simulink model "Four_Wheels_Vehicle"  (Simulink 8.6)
settings: Solver=ode45  StartTime=0.0  StopTime=20  RelTol=1e-3
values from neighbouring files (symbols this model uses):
  beta = 1    [Vehicle_Parameters.m]
  g = 9.81    [Vehicle_Parameters.m]
  H_CoG = 0.700    (= 0.7)    [Vehicle_Parameters.m]
  Hearo = 0.750    (= 0.75)    [Vehicle_Parameters.m]
  Iz = 2480    [Vehicle_Parameters.m]
  Jw = 2.166    [Vehicle_Parameters.m]
  L = 10    [Vehicle_Parameters.m]
  Lf = 1.180    (= 1.18)    [Vehicle_Parameters.m]
  Lr = 1.770    (= 1.77)    [Vehicle_Parameters.m]
  Lw = 1.880    (= 1.88)    [Vehicle_Parameters.m]
  m = 1500    [Vehicle_Parameters.m]
  miu = 0.85    [Vehicle_Parameters.m]
  reff = 0.380    (= 0.38)    [Vehicle_Parameters.m]
undefined symbols (not defined in the file or in its folder): DiscIntNeverNeededParam, Init, Ki, Kp, LowerLimit, sigbuilder_block, Ts, UpperLimit
libraries: simulink x15, powerlib_extras x3
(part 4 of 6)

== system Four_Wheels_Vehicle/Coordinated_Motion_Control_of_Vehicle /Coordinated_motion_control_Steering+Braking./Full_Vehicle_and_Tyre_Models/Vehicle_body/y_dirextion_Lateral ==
  note: y_dirextion_Lateral
  Fx_FL : Inport
  Fx_FR : Inport  Port=2
  Fy_FL : Inport  Port=3
  Fy_FR : Inport  Port=4
  Fy_RL : Inport  Port=5
  Fy_RR : Inport  Port=6
  Steering_Ang. : Inport  Port=7
  yaw_rate : Inport  Port=8
  x_Vel : Inport  Port=9
  1/m : Gain  Gain=1/1750
  Add1 : Sum
  Add12 : Sum
  Add15 : Sum  Inputs=++++
  Add2 : Sum  Inputs=+-
  Product1 : Product
  Product13 : Product
  Product3 : Product
  Vx0 : Integrator  UpperSaturationLimit=50/3.6  LowerSaturationLimit=eps
  cos_deltaw2 : Fcn  Expr=cos(u)
  sin_deltaw2 : Fcn  Expr=sin(u)
  y_Vel : Outport
  y total force : Outport  Port=2
  dy : Outport  Port=3
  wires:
  Steering_Ang./1 -> sin_deltaw2/1, cos_deltaw2/1
  Add12/1 -> Product13/1
  sin_deltaw2/1 -> Product13/2
  Add15/1 -> 1/m/1, y total force/1
  1/m/1 -> Add2/1
  Vx0/1 -> y_Vel/1
  Add1/1 -> Product1/1
  cos_deltaw2/1 -> Product1/2
  yaw_rate/1 -> Product3/1
  x_Vel/1 -> Product3/2
  Product3/1 -> Add2/2
  Fy_FL/1 -> Add1/1
  Fy_FR/1 -> Add1/2
  Fx_FL/1 -> Add12/1
  Fx_FR/1 -> Add12/2
  Product1/1 -> Add15/2
  Product13/1 -> Add15/1
  Fy_RR/1 -> Add15/4
  Fy_RL/1 -> Add15/3
  Add2/1 -> dy/1, Vx0/1

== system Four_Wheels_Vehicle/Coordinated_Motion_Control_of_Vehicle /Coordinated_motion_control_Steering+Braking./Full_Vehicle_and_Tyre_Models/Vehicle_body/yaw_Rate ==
  note: yaw_Rate_and_z_torque
  Fx_FL : Inport
  Fx_FR : Inport  Port=2
  Fy_FL : Inport  Port=3
  Fy_FR : Inport  Port=4
  Fx_RL : Inport  Port=5
  Fx_RR : Inport  Port=6
  Fy_RL : Inport  Port=7
  Fy_RR : Inport  Port=8
  Steering_Ang. : Inport  Port=9
  1/Iz : Gain  Gain=1/Iz
  Add1 : Sum  Inputs=-+
  Add10 : Sum  Inputs=+++++-
  Add2 : Sum
  Add3 : Sum  Inputs=-+
  Add4 : Sum
  Add5 : Sum  Inputs=-+
  Add6 : Sum
  Integrator1 : Integrator  InitialCondition=eps  UpperSaturationLimit=50/3.6  LowerSaturationLimit=eps  ShowSaturationPort=on
  Lf : Constant  Value=Lf
  Lr : Constant  Value=Lr
  Lw/2 : Constant  Value=Lw/2
  Product{1..9,13} (10 alike) : Product
  Stop Simulation1 : Stop
  cosdeltaw1 : Fcn  Expr=cos(u)
  sindeltaw1 : Fcn  Expr=sin(u)
  yaw_rate : Outport
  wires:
  Steering_Ang./1 -> cosdeltaw1/1, sindeltaw1/1
  Add4/1 -> Product1/1
  sindeltaw1/1 -> Product6/1, Product1/2
  Lf/1 -> Product3/2, Product13/1
  Add1/1 -> Product4/1
  cosdeltaw1/1 -> Product7/2, Product4/2
  Lw/2/1 -> Product5/2, Product2/2, Product9/2
  Lr/1 -> Product8/2
  Product3/1 -> Add10/1
  1/Iz/1 -> Integrator1/1
  Integrator1/1 -> yaw_rate/1
  Integrator1/2 -> Stop Simulation1/1
  Product1/1 -> Product3/1
  Product4/1 -> Product2/1
  Add2/1 -> Product7/1
  Add5/1 -> Product9/1
  Add6/1 -> Product8/1
  Product13/1 -> Add10/2
  Product7/1 -> Product13/2
  Product2/1 -> Add10/3
  Product8/1 -> Add10/6
  Product9/1 -> Add10/5
  Product5/1 -> Add10/4
  Product6/1 -> Product5/1
  Add3/1 -> Product6/2
  Add10/1 -> 1/Iz/1
  Fy_FR/1 -> Add2/2, Add3/1
  Fy_FL/1 -> Add3/2, Add2/1
  Fx_FL/1 -> Add4/1, Add1/1
  Fx_FR/1 -> Add4/2, Add1/2
  Fx_RL/1 -> Add5/1
  Fx_RR/1 -> Add5/2
  Fy_RL/1 -> Add6/1
  Fy_RR/1 -> Add6/2

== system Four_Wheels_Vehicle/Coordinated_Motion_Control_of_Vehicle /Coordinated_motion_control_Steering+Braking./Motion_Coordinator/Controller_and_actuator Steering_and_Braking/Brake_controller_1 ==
  Reference_Sideslip_1 : Inport
  Feedback_Sideslip_1 : Inport  Port=2
  Add1 : Sum
  Brake_Actuator_1 : Subsystem
  Brake_controller_1 : Subsystem
  Ramp : simulink/Sources/Ramp  slope=3  start=1  X0=0
  Sideslip_angle : Scope  NumInputPorts=2
  x_seitch2 : ManualSwitch  CurrentSetting=0
  Mzc_1 : Outport
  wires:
  Brake_Actuator_1/1(output) -> x_seitch2/2
  Ramp/1 -> x_seitch2/1
  Feedback_Sideslip_1/1 -> Sideslip_angle/2, Brake_controller_1/2(Feedback)
  Brake_controller_1/2(Sideslip_Ang1) -> Brake_Actuator_1/1(input)
  Reference_Sideslip_1/1 -> Add1/1, Sideslip_angle/1, Brake_controller_1/1(Reference)
  Add1/1 -> Mzc_1/1
  x_seitch2/1 -> Add1/2

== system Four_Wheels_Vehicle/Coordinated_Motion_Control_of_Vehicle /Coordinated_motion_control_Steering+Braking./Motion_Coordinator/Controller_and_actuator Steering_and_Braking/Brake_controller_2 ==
  Reference_Sideslip_2 : Inport
  Feedback_Sideslip_2 : Inport  Port=2
  Add1 : Sum
  Brake_Actuator_2 : Subsystem
  Brake_controller_2 : Subsystem
  Ramp : simulink/Sources/Ramp  slope=3  start=1  X0=0
  Sideslip_angle : Scope  NumInputPorts=2
  x_seitch2 : ManualSwitch  CurrentSetting=0
  Mzc_2 : Outport
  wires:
  x_seitch2/1 -> Add1/2
  Add1/1 -> Mzc_2/1
  Reference_Sideslip_2/1 -> Brake_controller_2/1(Reference), Sideslip_angle/1, Add1/1
  Brake_controller_2/2(Sideslip_Ang1) -> Brake_Actuator_2/1(input)
  Feedback_Sideslip_2/1 -> Brake_controller_2/2(Feedback), Sideslip_angle/2
  Ramp/1 -> x_seitch2/1
  Brake_Actuator_2/1(output) -> x_seitch2/2

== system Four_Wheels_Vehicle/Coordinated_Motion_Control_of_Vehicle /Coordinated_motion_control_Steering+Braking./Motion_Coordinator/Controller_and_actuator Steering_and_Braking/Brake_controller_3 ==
  Reference_Sideslip_3 : Inport
  Feedback_Sideslip_3 : Inport  Port=2
  Add1 : Sum
  Brake_Actuator_3 : Subsystem
  Brake_controller_3 : Subsystem
  Ramp : simulink/Sources/Ramp  slope=3  start=1  X0=0
  Sideslip_angle : Scope  NumInputPorts=2
  x_seitch2 : ManualSwitch  CurrentSetting=0
  Mzc_3 : Outport
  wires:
  Brake_Actuator_3/1(output) -> x_seitch2/2
  Ramp/1 -> x_seitch2/1
  Feedback_Sideslip_3/1 -> Sideslip_angle/2, Brake_controller_3/2(Feedback)
  Brake_controller_3/2(Sideslip_Ang1) -> Brake_Actuator_3/1(input)
  Reference_Sideslip_3/1 -> Add1/1, Sideslip_angle/1, Brake_controller_3/1(Reference)
  Add1/1 -> Mzc_3/1
  x_seitch2/1 -> Add1/2

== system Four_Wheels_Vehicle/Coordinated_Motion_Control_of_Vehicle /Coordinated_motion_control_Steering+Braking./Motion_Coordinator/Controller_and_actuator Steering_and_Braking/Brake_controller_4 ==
  Reference_Sideslip_4 : Inport
  Feedback_Sideslip_4 : Inport  Port=2
  Add1 : Sum
  Brake_Actuator_4 : Subsystem
  Brake_controller_4 : Subsystem
  Ramp : simulink/Sources/Ramp  slope=3  start=1  X0=0
  Sideslip_angle : Scope  NumInputPorts=2
  x_seitch2 : ManualSwitch  CurrentSetting=0
  Mzc_4 : Outport
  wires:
  x_seitch2/1 -> Add1/2
  Add1/1 -> Mzc_4/1
  Reference_Sideslip_4/1 -> Brake_controller_4/1(Reference), Sideslip_angle/1, Add1/1
  Brake_controller_4/2(Sideslip_Ang1) -> Brake_Actuator_4/1(input)
  Feedback_Sideslip_4/1 -> Brake_controller_4/2(Feedback), Sideslip_angle/2
  Ramp/1 -> x_seitch2/1
  Brake_Actuator_4/1(output) -> x_seitch2/2

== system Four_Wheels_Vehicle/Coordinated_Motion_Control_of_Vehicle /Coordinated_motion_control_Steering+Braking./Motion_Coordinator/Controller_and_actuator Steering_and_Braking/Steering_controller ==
  StteringAng : Inport
  Reference_Steering : Inport  Port=2
  Feedback_Steering : Inport  Port=3
  Add : Sum
  Steering_Actuator : Subsystem
  Steering_controller : Subsystem
  x_seitch1 : ManualSwitch  CurrentSetting=0
  yaw_comparsion : Scope  NumInputPorts=2
  f : Outport
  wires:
  Add/1 -> f/1
  Feedback_Steering/1 -> yaw_comparsion/2, Steering_controller/2(Feedback)
  Steering_Actuator/1(output) -> x_seitch1/2
  Steering_controller/2(Steering_Ang1) -> Steering_Actuator/1(input)
  x_seitch1/1 -> Add/2
  StteringAng/1 -> Add/1
  Reference_Steering/1 -> x_seitch1/1, Steering_controller/1(Reference), yaw_comparsion/1

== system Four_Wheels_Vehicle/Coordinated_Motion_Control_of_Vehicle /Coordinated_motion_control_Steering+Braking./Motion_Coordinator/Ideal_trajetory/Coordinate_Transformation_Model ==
  note: vehicle heading
  delta_steer (rad) : Inport
  v_x (m/s) : Inport  Port=2
  1/L : Gain  Gain=1/L
  Beta : Scope
  Beta1 : Scope
  Divide : Product  Inputs=*/
  Gain : Gain  Gain=L/2
  Gain1 : Gain  Gain=0.1
  Gain2 : Gain  Gain=0.1
  Gain4 : Gain  Gain=0.345
  Ground : Ground
  Integrator : Integrator
  Integrator1 : Integrator  LimitOutput=on  UpperSaturationLimit=0
  Integrator2 : Integrator
  Product{,1,3..4} (4 alike) : Product
  Sideslip_angle : Scope
  Subtract : Sum  Inputs=+-
  Sum : Sum  Inputs=|+-
  Sum1 : Sum  Inputs=|++
  Terminator : Terminator
  Trigonometric Function : Trigonometry  Operator=cos
  Trigonometric Function1 : Trigonometry
  Trigonometric Function2 : Trigonometry  Operator=atan
  Trigonometric Function3 : Trigonometry  Operator=tan
  steerVsYawrate1 : Scope  NumInputPorts=3
  steerVsYawrate2 : Scope  NumInputPorts=3
  yaw_rate : Product
  X-position : Outport
  Y-position : Outport  Port=2
  yaw_Rate : Outport  Port=3
  Sideslip_beta : Outport  Port=4
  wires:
  Subtract/1 -> Beta/1
  Gain4/1 -> Divide/1, Integrator1/1, steerVsYawrate2/3
  Trigonometric Function2/1 -> Subtract/1, Sideslip_beta/1, Sideslip_angle/1
  Gain2/1 -> Integrator2/1
  Gain1/1 -> Trigonometric Function1/1, steerVsYawrate1/3, Trigonometric Function/1
  delta_steer (rad)/1 -> yaw_rate/2
  Divide/1 -> Trigonometric Function2/1
  Trigonometric Function3/1 -> Terminator/1
  Ground/1 -> Trigonometric Function3/1
  Product4/1 -> Sum1/2
  Product3/1 -> Sum/2
  Gain/1 -> Product4/1, Product3/1  "L/2*psi-dot"
  Sum1/1 -> Gain4/1  "v_Y (m/s)"
  Sum/1 -> Divide/2, Integrator/1, steerVsYawrate2/2  "v_X (m/s)"
  1/L/1 -> yaw_rate/1  "v_x / L"
  yaw_rate/1 -> Gain2/1, yaw_Rate/1, Subtract/2, Beta1/1, Gain/1, steerVsYawrate2/1
  v_x (m/s)/1 -> 1/L/1, Product1/1, Product/1  "v_x (m/s)"
  Integrator1/1 -> Y-position/1, steerVsYawrate1/2
  Integrator/1 -> X-position/1, steerVsYawrate1/1
  Integrator2/1 -> Gain1/1  "yaw_heading (rad)"
  Trigonometric Function1/1 -> Product3/2, Product/2  "sin(psi)"
  Trigonometric Function/1 -> Product4/2, Product1/2  "cos(psi)"
  Product1/1 -> Sum/1
  Product/1 -> Sum1/1

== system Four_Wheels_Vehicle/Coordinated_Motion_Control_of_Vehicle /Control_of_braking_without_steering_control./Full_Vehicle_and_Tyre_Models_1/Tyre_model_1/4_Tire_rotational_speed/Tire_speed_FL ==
  Tb_FL_1 : Inport
  Td_FL_1 : Inport  Port=2
  Fx_FL_1 : Inport  Port=3
  1/Jw : Gain  Gain=1/Jw
  Add22 : Sum  Inputs=-+
  Add23 : Sum  Inputs=+-
  Product27 : Product
  Stop Simulation5 : Stop
  Vx0 : Integrator  InitialCondition=14.3  UpperSaturationLimit=50/3.6  LowerSaturationLimit=eps  ShowSaturationPort=on
  reff : Constant  Value=reff
  Omega_FL_1 : Outport
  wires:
  Fx_FL_1/1 -> Product27/1
  Vx0/2 -> Stop Simulation5/1
  Vx0/1 -> Omega_FL_1/1
  Add23/1 -> 1/Jw/1
  Add22/1 -> Add23/1
  Product27/1 -> Add23/2
  reff/1 -> Product27/2
  Td_FL_1/1 -> Add22/2
  Tb_FL_1/1 -> Add22/1
  1/Jw/1 -> Vx0/1

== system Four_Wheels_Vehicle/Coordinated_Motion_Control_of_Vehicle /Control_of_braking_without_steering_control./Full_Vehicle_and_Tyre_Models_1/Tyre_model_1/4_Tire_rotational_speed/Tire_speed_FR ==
  Tb_FR_1 : Inport
  Td_FR_1 : Inport  Port=2
  Fx_FR_1 : Inport  Port=3
  1/Jw : Gain  Gain=1/Jw
  Add1 : Sum  Inputs=+-
  Add24 : Sum  Inputs=-+
  Product1 : Product
  Stop Simulation6 : Stop
  Vx1 : Integrator  InitialCondition=14.3  UpperSaturationLimit=50/3.6  LowerSaturationLimit=eps  ShowSaturationPort=on
  reff : Constant  Value=reff
  Omega_FR_1 : Outport
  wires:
  Vx1/1 -> Omega_FR_1/1
  Vx1/2 -> Stop Simulation6/1
  Fx_FR_1/1 -> Product1/1
  reff/1 -> Product1/2
  Tb_FR_1/1 -> Add24/1
  Td_FR_1/1 -> Add24/2
  Add24/1 -> Add1/1
  1/Jw/1 -> Vx1/1
  Add1/1 -> 1/Jw/1
  Product1/1 -> Add1/2

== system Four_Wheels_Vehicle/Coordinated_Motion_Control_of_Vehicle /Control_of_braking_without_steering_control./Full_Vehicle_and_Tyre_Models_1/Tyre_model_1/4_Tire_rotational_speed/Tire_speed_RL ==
  Tb_RL_1 : Inport
  Td_RL_1 : Inport  Port=2
  Fx_RL_1 : Inport  Port=3
  1/Jw : Gain  Gain=1/Jw
  Add2 : Sum  Inputs=--
  Add22 : Sum  Inputs=-+
  Product2 : Product
  Stop Simulation7 : Stop
  Vx2 : Integrator  InitialCondition=14.3  UpperSaturationLimit=50/3.6  LowerSaturationLimit=eps  ShowSaturationPort=on
  reff : Constant  Value=reff
  Omega_RL_1 : Outport
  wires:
  Td_RL_1/1 -> Add22/2
  Tb_RL_1/1 -> Add22/1
  Add22/1 -> Add2/1
  Add2/1 -> 1/Jw/1
  Product2/1 -> Add2/2
  reff/1 -> Product2/2
  Vx2/1 -> Omega_RL_1/1
  Vx2/2 -> Stop Simulation7/1
  1/Jw/1 -> Vx2/1
  Fx_RL_1/1 -> Product2/1

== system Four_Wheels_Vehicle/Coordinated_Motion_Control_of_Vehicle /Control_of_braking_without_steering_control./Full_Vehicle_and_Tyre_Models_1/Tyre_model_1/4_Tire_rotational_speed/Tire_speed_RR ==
  Tb_RR_1 : Inport
  Td_RR_1 : Inport  Port=2
  Fx_RR_1 : Inport  Port=3
  1/Jw : Gain  Gain=1/Jw
  Add22 : Sum  Inputs=-+
  Add3 : Sum  Inputs=--
  Product3 : Product
  Stop Simulation8 : Stop
  Vx3 : Integrator  InitialCondition=14.3  UpperSaturationLimit=50/3.6  LowerSaturationLimit=eps  ShowSaturationPort=on
  reff : Constant  Value=reff
  Omega_RR_1 : Outport
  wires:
  Td_RR_1/1 -> Add22/2
  Tb_RR_1/1 -> Add22/1
  Add22/1 -> Add3/1
  Product3/1 -> Add3/2
  Fx_RR_1/1 -> Product3/1
  reff/1 -> Product3/2
  1/Jw/1 -> Vx3/1
  Add3/1 -> 1/Jw/1
  Vx3/2 -> Stop Simulation8/1
  Vx3/1 -> Omega_RR_1/1

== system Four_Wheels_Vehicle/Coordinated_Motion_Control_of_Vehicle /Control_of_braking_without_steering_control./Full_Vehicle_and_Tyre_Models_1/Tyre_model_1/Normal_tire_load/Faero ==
  note: Air Drag Faero
  Vx : Inport
  AirDragConst1 : Inport  Port=2
  FrontalArea1 : Inport  Port=3
  Airdensity : Inport  Port=4
  windVelocity : Inport  Port=5
  Add : Sum
  Constant : Constant  Value=0.5
  Math Function : Math  Operator=square
  Product : Product  Inputs=5
  Faero : Outport
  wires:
  Vx/1 -> Add/2
  Airdensity/1 -> Product/3
  AirDragConst1/1 -> Product/1
  Product/1 -> Faero/1
  Math Function/1 -> Product/5
  Add/1 -> Math Function/1
  windVelocity/1 -> Add/1
  Constant/1 -> Product/4
  FrontalArea1/1 -> Product/2

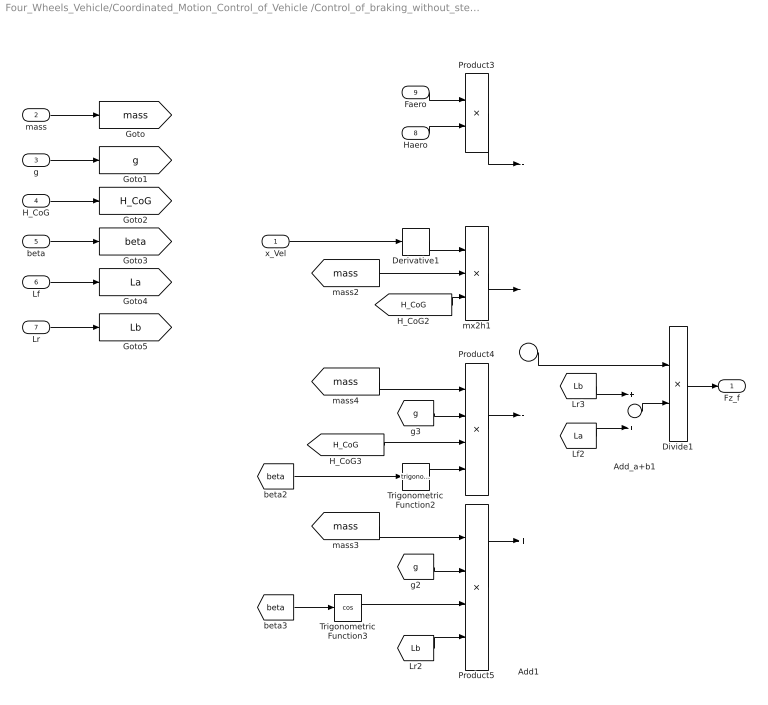
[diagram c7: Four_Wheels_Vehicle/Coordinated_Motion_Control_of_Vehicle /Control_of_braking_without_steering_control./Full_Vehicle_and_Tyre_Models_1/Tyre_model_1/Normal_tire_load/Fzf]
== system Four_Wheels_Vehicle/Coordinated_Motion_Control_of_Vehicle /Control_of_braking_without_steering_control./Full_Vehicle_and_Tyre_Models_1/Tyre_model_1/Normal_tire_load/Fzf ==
  x_Vel : Inport
  mass : Inport  Port=2
  g : Inport  Port=3
  H_CoG : Inport  Port=4
  beta : Inport  Port=5
  Lf : Inport  Port=6
  Lr : Inport  Port=7
  Haero : Inport  Port=8
  Faero : Inport  Port=9
  Add1 : Sum  Inputs=---+
  Add_a+b1 : Sum
  Derivative1 : Derivative
  Divide1 : Product  Inputs=*/
  Product3 : Product
  Product4 : Product  Inputs=4
  Product5 : Product  Inputs=4
  Trigonometric Function2 : Trigonometry
  Trigonometric Function3 : Trigonometry  Operator=cos
  mx2h1 : Product  Inputs=3
  Fz_f : Outport
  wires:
  Lf/1 -> [La]
  mass/1 -> [mass]
  Haero/1 -> Product3/2
  Faero/1 -> Product3/1
  Lr/1 -> [Lb]
  beta/1 -> [beta]
  H_CoG/1 -> [H_CoG]
  g/1 -> [g]
  [g] -> Product5/2
  [mass] -> mx2h1/2
  [g] -> Product4/2
  [mass] -> Product4/1
  x_Vel/1 -> Derivative1/1
  Divide1/1 -> Fz_f/1
  Add_a+b1/1 -> Divide1/2
  Add1/1 -> Divide1/1
  Product5/1 -> Add1/4
  Product4/1 -> Add1/3
  mx2h1/1 -> Add1/2
  Product3/1 -> Add1/1
  [La] -> Add_a+b1/2
  [Lb] -> Add_a+b1/1
  [Lb] -> Product5/4
  Trigonometric Function3/1 -> Product5/3
  [mass] -> Product5/1
  Trigonometric Function2/1 -> Product4/4
  [H_CoG] -> Product4/3
  [beta] -> Trigonometric Function3/1
  [beta] -> Trigonometric Function2/1
  [H_CoG] -> mx2h1/3
  Derivative1/1 -> mx2h1/1

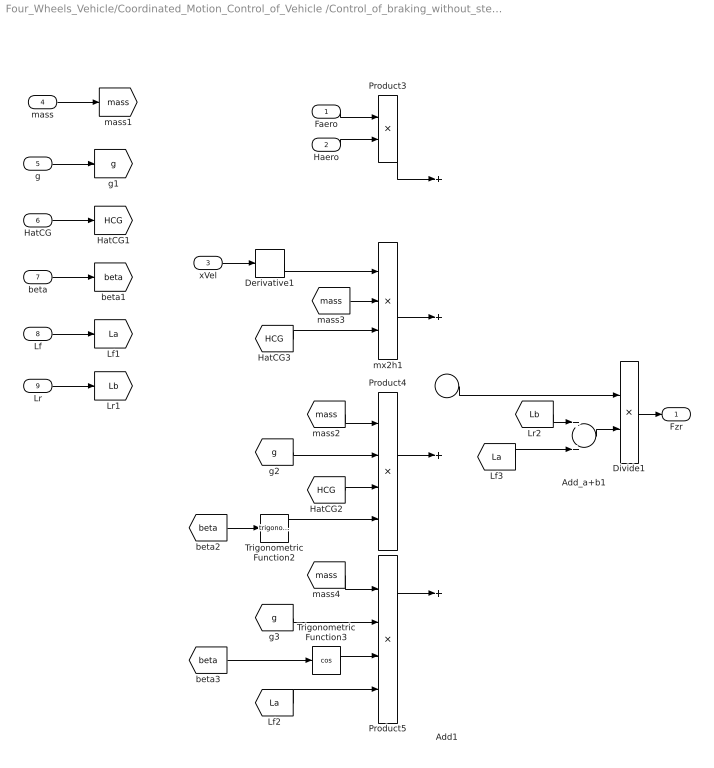
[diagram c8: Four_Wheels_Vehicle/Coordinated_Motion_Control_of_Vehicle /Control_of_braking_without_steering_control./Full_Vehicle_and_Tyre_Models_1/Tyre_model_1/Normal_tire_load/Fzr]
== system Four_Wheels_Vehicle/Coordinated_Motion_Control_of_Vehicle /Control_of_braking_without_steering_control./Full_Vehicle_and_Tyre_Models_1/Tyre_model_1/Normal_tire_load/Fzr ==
  Faero : Inport
  Haero : Inport  Port=2
  xVel : Inport  Port=3
  mass : Inport  Port=4
  g : Inport  Port=5
  HatCG : Inport  Port=6
  beta : Inport  Port=7
  Lf : Inport  Port=8
  Lr : Inport  Port=9
  Add1 : Sum  Inputs=++++
  Add_a+b1 : Sum
  Derivative1 : Derivative
  Divide1 : Product  Inputs=*/
  Product3 : Product
  Product4 : Product  Inputs=4
  Product5 : Product  Inputs=4
  Trigonometric Function2 : Trigonometry
  Trigonometric Function3 : Trigonometry  Operator=cos
  mx2h1 : Product  Inputs=3
  Fzr : Outport
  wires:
  Faero/1 -> Product3/1
  Haero/1 -> Product3/2
  Derivative1/1 -> mx2h1/1
  [HCG] -> mx2h1/3
  [beta] -> Trigonometric Function2/1
  [beta] -> Trigonometric Function3/1
  [HCG] -> Product4/3
  Trigonometric Function2/1 -> Product4/4
  [mass] -> Product5/1
  Trigonometric Function3/1 -> Product5/3
  [La] -> Product5/4
  [Lb] -> Add_a+b1/1
  [La] -> Add_a+b1/2
  Product3/1 -> Add1/1
  mx2h1/1 -> Add1/2
  Product4/1 -> Add1/3
  Product5/1 -> Add1/4
  Add1/1 -> Divide1/1
  Add_a+b1/1 -> Divide1/2
  Divide1/1 -> Fzr/1
  xVel/1 -> Derivative1/1
  mass/1 -> [mass]
  [mass] -> Product4/1
  g/1 -> [g]
  [g] -> Product4/2
  [mass] -> mx2h1/2
  [g] -> Product5/2
  HatCG/1 -> [HCG]
  beta/1 -> [beta]
  Lf/1 -> [La]
  Lr/1 -> [Lb]

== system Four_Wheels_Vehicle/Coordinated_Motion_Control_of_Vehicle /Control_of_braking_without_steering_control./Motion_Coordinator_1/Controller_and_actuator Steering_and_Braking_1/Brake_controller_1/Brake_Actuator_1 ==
  input : Inport
  Actuator : Subsystem
  Cut_off_frequency : Constant  Value=10  SampleTime=-1
  output : Outport
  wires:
  Cut_off_frequency/1 -> Actuator/2(fre)
  Actuator/1(out) -> output/1
  input/1 -> Actuator/1(In1)

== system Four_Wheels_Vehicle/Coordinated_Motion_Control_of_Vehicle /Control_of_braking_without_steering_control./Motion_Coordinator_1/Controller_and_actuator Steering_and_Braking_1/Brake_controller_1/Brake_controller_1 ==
  Reference : Inport
  Feedback : Inport  Port=2
  Controller : Subsystem  AncestorBlock=|  DialogController=POWERSYS.PowerSysDialog
      | powerlib_extras/Discrete 
      | Control Blocks/Discrete
      | PI Controller
  Controller1 : Subsystem  AncestorBlock=|  DialogController=POWERSYS.PowerSysDialog
      | powerlib_extras/Discrete 
      | Control Blocks/Discrete
      | PI Controller
  Scope : Scope
  Scope1 : Scope
  Scope2 : Scope  NumInputPorts=2
  Sum1 : Sum  Inputs=-+
  Sum2 : Sum
  Sideslip_Ang : Outport
  Sideslip_Ang1 : Outport  Port=2
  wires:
  Sum2/1 -> Sideslip_Ang1/1, Scope2/2
  Reference/1 -> Sum1/2, Controller1/1(Error)
  Controller1/1(Out) -> Sum2/2
  Feedback/1 -> Sum1/1
  Sum1/1 -> Scope/1, Controller/1(Error)
  Controller/1(Out) -> Sideslip_Ang/1, Scope2/1, Sum2/1, Scope1/1

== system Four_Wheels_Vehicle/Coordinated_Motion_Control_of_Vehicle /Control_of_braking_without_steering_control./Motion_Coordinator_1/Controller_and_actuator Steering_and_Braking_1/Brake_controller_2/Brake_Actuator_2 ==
  input : Inport
  Actuator : Subsystem
  Cut_off_frequency : Constant  Value=10  SampleTime=-1
  output : Outport
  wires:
  input/1 -> Actuator/1(In1)
  Actuator/1(out) -> output/1
  Cut_off_frequency/1 -> Actuator/2(fre)

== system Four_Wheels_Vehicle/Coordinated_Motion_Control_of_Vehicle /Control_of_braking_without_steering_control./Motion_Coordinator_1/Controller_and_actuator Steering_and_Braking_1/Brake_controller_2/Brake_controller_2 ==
  Reference : Inport
  Feedback : Inport  Port=2
  Controller : Subsystem  AncestorBlock=|  DialogController=POWERSYS.PowerSysDialog
      | powerlib_extras/Discrete 
      | Control Blocks/Discrete
      | PI Controller
  Controller1 : Subsystem  AncestorBlock=|  DialogController=POWERSYS.PowerSysDialog
      | powerlib_extras/Discrete 
      | Control Blocks/Discrete
      | PI Controller
  Scope : Scope
  Scope1 : Scope
  Scope2 : Scope  NumInputPorts=2
  Sum1 : Sum  Inputs=-+
  Sum2 : Sum
  Sideslip_Ang : Outport
  Sideslip_Ang1 : Outport  Port=2
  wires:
  Controller/1(Out) -> Scope1/1, Sum2/1, Scope2/1, Sideslip_Ang/1
  Sum1/1 -> Controller/1(Error), Scope/1
  Feedback/1 -> Sum1/1
  Controller1/1(Out) -> Sum2/2
  Reference/1 -> Controller1/1(Error), Sum1/2
  Sum2/1 -> Scope2/2, Sideslip_Ang1/1

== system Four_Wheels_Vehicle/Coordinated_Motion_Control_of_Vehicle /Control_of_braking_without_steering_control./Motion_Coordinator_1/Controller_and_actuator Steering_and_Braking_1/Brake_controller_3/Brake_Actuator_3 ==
  input : Inport
  Actuator : Subsystem
  Cut_off_frequency : Constant  Value=10  SampleTime=-1
  output : Outport
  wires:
  Cut_off_frequency/1 -> Actuator/2(fre)
  Actuator/1(out) -> output/1
  input/1 -> Actuator/1(In1)

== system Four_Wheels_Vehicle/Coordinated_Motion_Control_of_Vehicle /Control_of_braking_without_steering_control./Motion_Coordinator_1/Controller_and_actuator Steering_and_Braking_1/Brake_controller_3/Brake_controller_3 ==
  Reference : Inport
  Feedback : Inport  Port=2
  Controller : Subsystem  AncestorBlock=|  DialogController=POWERSYS.PowerSysDialog
      | powerlib_extras/Discrete 
      | Control Blocks/Discrete
      | PI Controller
  Controller1 : Subsystem  AncestorBlock=|  DialogController=POWERSYS.PowerSysDialog
      | powerlib_extras/Discrete 
      | Control Blocks/Discrete
      | PI Controller
  Scope : Scope
  Scope1 : Scope
  Scope2 : Scope  NumInputPorts=2
  Sum1 : Sum  Inputs=-+
  Sum2 : Sum
  Sideslip_Ang : Outport
  Sideslip_Ang1 : Outport  Port=2
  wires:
  Sum2/1 -> Sideslip_Ang1/1, Scope2/2
  Reference/1 -> Sum1/2, Controller1/1(Error)
  Controller1/1(Out) -> Sum2/2
  Feedback/1 -> Sum1/1
  Sum1/1 -> Scope/1, Controller/1(Error)
  Controller/1(Out) -> Sideslip_Ang/1, Scope2/1, Sum2/1, Scope1/1

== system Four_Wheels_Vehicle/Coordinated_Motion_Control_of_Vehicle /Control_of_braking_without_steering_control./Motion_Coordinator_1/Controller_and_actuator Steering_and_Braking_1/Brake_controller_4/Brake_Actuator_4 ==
  input : Inport
  Actuator : Subsystem
  Cut_off_frequency : Constant  Value=10  SampleTime=-1
  output : Outport
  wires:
  input/1 -> Actuator/1(In1)
  Actuator/1(out) -> output/1
  Cut_off_frequency/1 -> Actuator/2(fre)

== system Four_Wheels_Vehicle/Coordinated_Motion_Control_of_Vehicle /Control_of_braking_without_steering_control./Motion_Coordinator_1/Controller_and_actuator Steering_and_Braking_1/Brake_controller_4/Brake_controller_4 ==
  Reference : Inport
  Feedback : Inport  Port=2
  Controller : Subsystem  AncestorBlock=|  DialogController=POWERSYS.PowerSysDialog
      | powerlib_extras/Discrete 
      | Control Blocks/Discrete
      | PI Controller
  Controller1 : Subsystem  AncestorBlock=|  DialogController=POWERSYS.PowerSysDialog
      | powerlib_extras/Discrete 
      | Control Blocks/Discrete
      | PI Controller
  Scope : Scope
  Scope1 : Scope
  Scope2 : Scope  NumInputPorts=2
  Sum1 : Sum  Inputs=-+
  Sum2 : Sum
  Sideslip_Ang : Outport
  Sideslip_Ang1 : Outport  Port=2
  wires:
  Controller/1(Out) -> Scope1/1, Sum2/1, Scope2/1, Sideslip_Ang/1
  Sum1/1 -> Controller/1(Error), Scope/1
  Feedback/1 -> Sum1/1
  Controller1/1(Out) -> Sum2/2
  Reference/1 -> Controller1/1(Error), Sum1/2
  Sum2/1 -> Scope2/2, Sideslip_Ang1/1

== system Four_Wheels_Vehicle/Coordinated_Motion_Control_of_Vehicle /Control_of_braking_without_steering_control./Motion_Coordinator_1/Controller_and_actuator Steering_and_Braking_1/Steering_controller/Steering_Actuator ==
  input : Inport
  Actuator : Subsystem
  Cut_off_frequency : Constant  Value=5  SampleTime=-1
  output : Outport
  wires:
  input/1 -> Actuator/1(In1)
  Actuator/1(out) -> output/1
  Cut_off_frequency/1 -> Actuator/2(fre)

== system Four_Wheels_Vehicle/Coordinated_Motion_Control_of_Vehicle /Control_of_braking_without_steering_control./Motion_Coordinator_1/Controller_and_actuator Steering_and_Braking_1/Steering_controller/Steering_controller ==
  Reference : Inport
  Feedback : Inport  Port=2
  Controller : Subsystem  AncestorBlock=|  DialogController=POWERSYS.PowerSysDialog
      | powerlib_extras/Discrete 
      | Control Blocks/Discrete
      | PI Controller
  Controller1 : Subsystem  AncestorBlock=|  DialogController=POWERSYS.PowerSysDialog
      | powerlib_extras/Discrete 
      | Control Blocks/Discrete
      | PI Controller
  Scope : Scope
  Scope1 : Scope
  Scope2 : Scope  NumInputPorts=2
  Scope3 : Scope  NumInputPorts=2
  Sum1 : Sum  Inputs=-+
  Sum2 : Sum
  Steering_Ang : Outport
  Steering_Ang1 : Outport  Port=2
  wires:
  Controller1/1(Out) -> Sum2/2
  Sum2/1 -> Steering_Ang1/1, Scope2/2, Scope3/1
  Controller/1(Out) -> Scope1/1, Steering_Ang/1, Scope2/1, Sum2/1
  Reference/1 -> Sum1/2, Controller1/1(Error), Scope3/2
  Sum1/1 -> Controller/1(Error), Scope/1
  Feedback/1 -> Sum1/1

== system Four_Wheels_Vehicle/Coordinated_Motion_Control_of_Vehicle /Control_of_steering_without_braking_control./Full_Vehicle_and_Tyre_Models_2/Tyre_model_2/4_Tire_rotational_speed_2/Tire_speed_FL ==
  Tb_FL_2 : Inport
  Td_FL_2 : Inport  Port=2
  Fx_FL_2 : Inport  Port=3
  1/Jw : Gain  Gain=1/Jw
  Add22 : Sum  Inputs=-+
  Add23 : Sum  Inputs=+-
  Product27 : Product
  Stop Simulation5 : Stop
  Vx0 : Integrator  InitialCondition=14.3  UpperSaturationLimit=50/3.6  LowerSaturationLimit=eps  ShowSaturationPort=on
  reff : Constant  Value=reff
  Omega_FL_2 : Outport
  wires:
  1/Jw/1 -> Vx0/1
  Tb_FL_2/1 -> Add22/1
  Td_FL_2/1 -> Add22/2
  reff/1 -> Product27/2
  Product27/1 -> Add23/2
  Add22/1 -> Add23/1
  Add23/1 -> 1/Jw/1
  Vx0/1 -> Omega_FL_2/1
  Vx0/2 -> Stop Simulation5/1
  Fx_FL_2/1 -> Product27/1

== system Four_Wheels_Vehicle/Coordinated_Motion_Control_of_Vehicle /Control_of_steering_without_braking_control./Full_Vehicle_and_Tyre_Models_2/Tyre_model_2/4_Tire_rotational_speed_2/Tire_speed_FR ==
  Tb_FR_2 : Inport
  Td_FR_2 : Inport  Port=2
  Fx_FR_2 : Inport  Port=3
  1/Jw : Gain  Gain=1/Jw
  Add1 : Sum  Inputs=+-
  Add24 : Sum  Inputs=-+
  Product1 : Product
  Stop Simulation6 : Stop
  Vx1 : Integrator  InitialCondition=14.3  UpperSaturationLimit=50/3.6  LowerSaturationLimit=eps  ShowSaturationPort=on
  reff : Constant  Value=reff
  Omega_FR_2 : Outport
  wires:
  Product1/1 -> Add1/2
  Add1/1 -> 1/Jw/1
  1/Jw/1 -> Vx1/1
  Add24/1 -> Add1/1
  Td_FR_2/1 -> Add24/2
  Tb_FR_2/1 -> Add24/1
  reff/1 -> Product1/2
  Fx_FR_2/1 -> Product1/1
  Vx1/2 -> Stop Simulation6/1
  Vx1/1 -> Omega_FR_2/1

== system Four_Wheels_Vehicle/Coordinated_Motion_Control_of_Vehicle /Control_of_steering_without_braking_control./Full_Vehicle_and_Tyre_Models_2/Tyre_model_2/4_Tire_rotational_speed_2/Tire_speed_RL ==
  Tb_RL_2 : Inport
  Td_RL_2 : Inport  Port=2
  Fx_RL_2 : Inport  Port=3
  1/Jw : Gain  Gain=1/Jw
  Add2 : Sum  Inputs=--
  Add22 : Sum  Inputs=-+
  Product2 : Product
  Stop Simulation7 : Stop
  Vx2 : Integrator  InitialCondition=14.3  UpperSaturationLimit=50/3.6  LowerSaturationLimit=eps  ShowSaturationPort=on
  reff : Constant  Value=reff
  Omega_RL_2 : Outport
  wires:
  Fx_RL_2/1 -> Product2/1
  1/Jw/1 -> Vx2/1
  Vx2/2 -> Stop Simulation7/1
  Vx2/1 -> Omega_RL_2/1
  reff/1 -> Product2/2
  Product2/1 -> Add2/2
  Add2/1 -> 1/Jw/1
  Add22/1 -> Add2/1
  Tb_RL_2/1 -> Add22/1
  Td_RL_2/1 -> Add22/2

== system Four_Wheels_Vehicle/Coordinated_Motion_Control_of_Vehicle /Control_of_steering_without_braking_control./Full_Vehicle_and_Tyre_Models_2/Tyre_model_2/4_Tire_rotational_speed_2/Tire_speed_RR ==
  Tb_RR_2 : Inport
  Td_RR_2 : Inport  Port=2
  Fx_RR_2 : Inport  Port=3
  1/Jw : Gain  Gain=1/Jw
  Add22 : Sum  Inputs=-+
  Add3 : Sum  Inputs=--
  Product3 : Product
  Stop Simulation8 : Stop
  Vx3 : Integrator  InitialCondition=14.3  UpperSaturationLimit=50/3.6  LowerSaturationLimit=eps  ShowSaturationPort=on
  reff : Constant  Value=reff
  Omega_RR_2 : Outport
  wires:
  Vx3/1 -> Omega_RR_2/1
  Vx3/2 -> Stop Simulation8/1
  Add3/1 -> 1/Jw/1
  1/Jw/1 -> Vx3/1
  reff/1 -> Product3/2
  Fx_RR_2/1 -> Product3/1
  Product3/1 -> Add3/2
  Add22/1 -> Add3/1
  Tb_RR_2/1 -> Add22/1
  Td_RR_2/1 -> Add22/2

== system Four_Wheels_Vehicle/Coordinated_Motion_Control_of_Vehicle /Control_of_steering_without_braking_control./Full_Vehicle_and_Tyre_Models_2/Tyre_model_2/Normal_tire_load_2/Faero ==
  note: Air Drag Faero
  Vx : Inport
  AirDragConst1 : Inport  Port=2
  FrontalArea1 : Inport  Port=3
  Airdensity : Inport  Port=4
  windVelocity : Inport  Port=5
  Add : Sum
  Constant : Constant  Value=0.5
  Math Function : Math  Operator=square
  Product : Product  Inputs=5
  Faero : Outport
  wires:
  FrontalArea1/1 -> Product/2
  Constant/1 -> Product/4
  windVelocity/1 -> Add/1
  Add/1 -> Math Function/1
  Math Function/1 -> Product/5
  Product/1 -> Faero/1
  AirDragConst1/1 -> Product/1
  Airdensity/1 -> Product/3
  Vx/1 -> Add/2

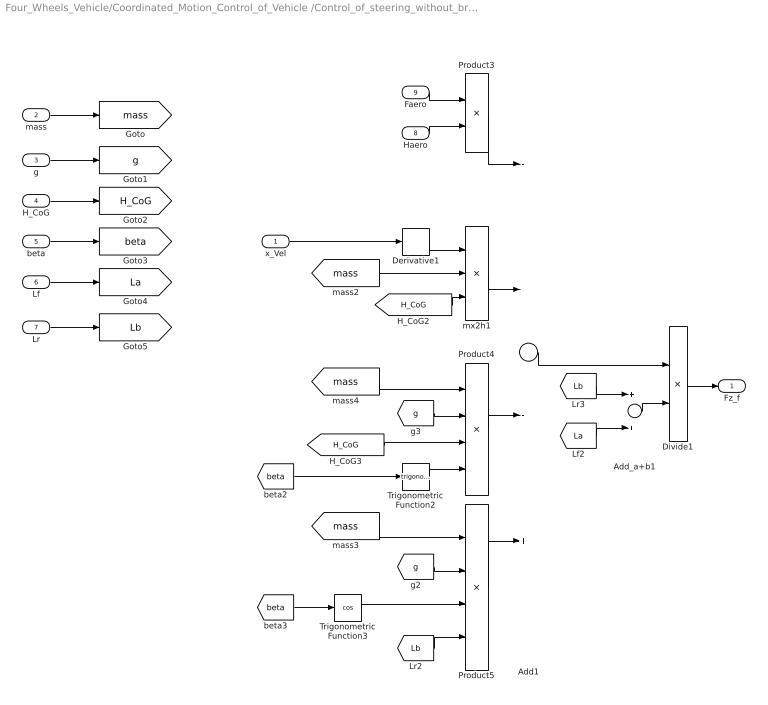
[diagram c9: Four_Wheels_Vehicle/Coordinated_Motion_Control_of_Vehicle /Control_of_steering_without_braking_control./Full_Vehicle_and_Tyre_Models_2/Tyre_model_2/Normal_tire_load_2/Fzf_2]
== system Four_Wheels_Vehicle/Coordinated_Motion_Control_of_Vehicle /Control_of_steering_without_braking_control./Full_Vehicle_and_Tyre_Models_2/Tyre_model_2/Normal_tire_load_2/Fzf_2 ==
  x_Vel : Inport
  mass : Inport  Port=2
  g : Inport  Port=3
  H_CoG : Inport  Port=4
  beta : Inport  Port=5
  Lf : Inport  Port=6
  Lr : Inport  Port=7
  Haero : Inport  Port=8
  Faero : Inport  Port=9
  Add1 : Sum  Inputs=---+
  Add_a+b1 : Sum
  Derivative1 : Derivative
  Divide1 : Product  Inputs=*/
  Product3 : Product
  Product4 : Product  Inputs=4
  Product5 : Product  Inputs=4
  Trigonometric Function2 : Trigonometry
  Trigonometric Function3 : Trigonometry  Operator=cos
  mx2h1 : Product  Inputs=3
  Fz_f : Outport
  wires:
  Derivative1/1 -> mx2h1/1
  [H_CoG] -> mx2h1/3
  [beta] -> Trigonometric Function2/1
  [beta] -> Trigonometric Function3/1
  [H_CoG] -> Product4/3
  Trigonometric Function2/1 -> Product4/4
  [mass] -> Product5/1
  Trigonometric Function3/1 -> Product5/3
  [Lb] -> Product5/4
  [Lb] -> Add_a+b1/1
  [La] -> Add_a+b1/2
  Product3/1 -> Add1/1
  mx2h1/1 -> Add1/2
  Product4/1 -> Add1/3
  Product5/1 -> Add1/4
  Add1/1 -> Divide1/1
  Add_a+b1/1 -> Divide1/2
  Divide1/1 -> Fz_f/1
  x_Vel/1 -> Derivative1/1
  [mass] -> Product4/1
  [g] -> Product4/2
  [mass] -> mx2h1/2
  [g] -> Product5/2
  g/1 -> [g]
  H_CoG/1 -> [H_CoG]
  beta/1 -> [beta]
  Lr/1 -> [Lb]
  Faero/1 -> Product3/1
  Haero/1 -> Product3/2
  mass/1 -> [mass]
  Lf/1 -> [La]

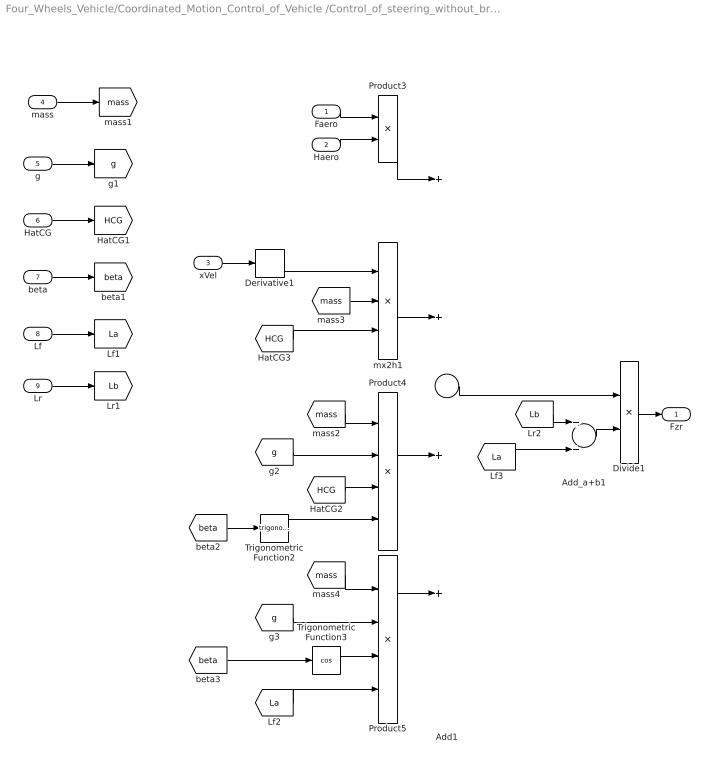
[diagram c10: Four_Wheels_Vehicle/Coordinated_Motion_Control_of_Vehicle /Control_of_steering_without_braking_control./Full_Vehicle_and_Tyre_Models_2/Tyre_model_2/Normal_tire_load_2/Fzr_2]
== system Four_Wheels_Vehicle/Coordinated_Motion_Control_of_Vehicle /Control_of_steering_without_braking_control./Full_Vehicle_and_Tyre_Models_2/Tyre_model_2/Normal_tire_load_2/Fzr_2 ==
  Faero : Inport
  Haero : Inport  Port=2
  xVel : Inport  Port=3
  mass : Inport  Port=4
  g : Inport  Port=5
  HatCG : Inport  Port=6
  beta : Inport  Port=7
  Lf : Inport  Port=8
  Lr : Inport  Port=9
  Add1 : Sum  Inputs=++++
  Add_a+b1 : Sum
  Derivative1 : Derivative
  Divide1 : Product  Inputs=*/
  Product3 : Product
  Product4 : Product  Inputs=4
  Product5 : Product  Inputs=4
  Trigonometric Function2 : Trigonometry
  Trigonometric Function3 : Trigonometry  Operator=cos
  mx2h1 : Product  Inputs=3
  Fzr : Outport
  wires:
  Lr/1 -> [Lb]
  Lf/1 -> [La]
  beta/1 -> [beta]
  HatCG/1 -> [HCG]
  [g] -> Product5/2
  [mass] -> mx2h1/2
  [g] -> Product4/2
  g/1 -> [g]
  [mass] -> Product4/1
  mass/1 -> [mass]
  xVel/1 -> Derivative1/1
  Divide1/1 -> Fzr/1
  Add_a+b1/1 -> Divide1/2
  Add1/1 -> Divide1/1
  Product5/1 -> Add1/4
  Product4/1 -> Add1/3
  mx2h1/1 -> Add1/2
  Product3/1 -> Add1/1
  [La] -> Add_a+b1/2
  [Lb] -> Add_a+b1/1
  [La] -> Product5/4
  Trigonometric Function3/1 -> Product5/3
  [mass] -> Product5/1
  Trigonometric Function2/1 -> Product4/4
  [HCG] -> Product4/3
  [beta] -> Trigonometric Function3/1
  [beta] -> Trigonometric Function2/1
  [HCG] -> mx2h1/3
  Derivative1/1 -> mx2h1/1
  Haero/1 -> Product3/2
  Faero/1 -> Product3/1

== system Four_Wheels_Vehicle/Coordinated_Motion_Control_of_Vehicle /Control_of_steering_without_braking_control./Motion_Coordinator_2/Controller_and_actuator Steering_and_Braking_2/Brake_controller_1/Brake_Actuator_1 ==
  input : Inport
  Actuator : Subsystem
  Cut_off_frequency : Constant  Value=10  SampleTime=-1
  output : Outport
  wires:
  input/1 -> Actuator/1(In1)
  Actuator/1(out) -> output/1
  Cut_off_frequency/1 -> Actuator/2(fre)

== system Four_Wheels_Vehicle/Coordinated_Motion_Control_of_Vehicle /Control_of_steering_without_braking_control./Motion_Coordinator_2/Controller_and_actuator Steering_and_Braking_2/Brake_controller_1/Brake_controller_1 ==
  Reference : Inport
  Feedback : Inport  Port=2
  Controller : Subsystem  AncestorBlock=|  DialogController=POWERSYS.PowerSysDialog
      | powerlib_extras/Discrete 
      | Control Blocks/Discrete
      | PI Controller
  Controller1 : Subsystem  AncestorBlock=|  DialogController=POWERSYS.PowerSysDialog
      | powerlib_extras/Discrete 
      | Control Blocks/Discrete
      | PI Controller
  Scope : Scope
  Scope1 : Scope
  Scope2 : Scope  NumInputPorts=2
  Sum1 : Sum  Inputs=-+
  Sum2 : Sum
  Sideslip_Ang : Outport
  Sideslip_Ang1 : Outport  Port=2
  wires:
  Controller/1(Out) -> Scope1/1, Sum2/1, Scope2/1, Sideslip_Ang/1
  Sum1/1 -> Controller/1(Error), Scope/1
  Feedback/1 -> Sum1/1
  Controller1/1(Out) -> Sum2/2
  Reference/1 -> Controller1/1(Error), Sum1/2
  Sum2/1 -> Scope2/2, Sideslip_Ang1/1

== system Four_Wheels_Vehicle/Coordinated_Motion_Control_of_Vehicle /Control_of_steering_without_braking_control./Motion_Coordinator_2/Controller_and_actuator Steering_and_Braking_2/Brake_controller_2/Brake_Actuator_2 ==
  input : Inport
  Actuator : Subsystem
  Cut_off_frequency : Constant  Value=10  SampleTime=-1
  output : Outport
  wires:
  Cut_off_frequency/1 -> Actuator/2(fre)
  Actuator/1(out) -> output/1
  input/1 -> Actuator/1(In1)

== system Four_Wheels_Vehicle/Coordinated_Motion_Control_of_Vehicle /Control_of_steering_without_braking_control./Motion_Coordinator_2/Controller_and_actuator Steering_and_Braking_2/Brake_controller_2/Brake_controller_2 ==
  Reference : Inport
  Feedback : Inport  Port=2
  Controller : Subsystem  AncestorBlock=|  DialogController=POWERSYS.PowerSysDialog
      | powerlib_extras/Discrete 
      | Control Blocks/Discrete
      | PI Controller
  Controller1 : Subsystem  AncestorBlock=|  DialogController=POWERSYS.PowerSysDialog
      | powerlib_extras/Discrete 
      | Control Blocks/Discrete
      | PI Controller
  Scope : Scope
  Scope1 : Scope
  Scope2 : Scope  NumInputPorts=2
  Sum1 : Sum  Inputs=-+
  Sum2 : Sum
  Sideslip_Ang : Outport
  Sideslip_Ang1 : Outport  Port=2
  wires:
  Sum2/1 -> Sideslip_Ang1/1, Scope2/2
  Reference/1 -> Sum1/2, Controller1/1(Error)
  Controller1/1(Out) -> Sum2/2
  Feedback/1 -> Sum1/1
  Sum1/1 -> Scope/1, Controller/1(Error)
  Controller/1(Out) -> Sideslip_Ang/1, Scope2/1, Sum2/1, Scope1/1

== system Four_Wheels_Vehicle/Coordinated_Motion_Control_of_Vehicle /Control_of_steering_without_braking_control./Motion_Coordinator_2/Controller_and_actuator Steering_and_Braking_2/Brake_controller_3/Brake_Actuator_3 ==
  input : Inport
  Actuator : Subsystem
  Cut_off_frequency : Constant  Value=10  SampleTime=-1
  output : Outport
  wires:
  input/1 -> Actuator/1(In1)
  Actuator/1(out) -> output/1
  Cut_off_frequency/1 -> Actuator/2(fre)

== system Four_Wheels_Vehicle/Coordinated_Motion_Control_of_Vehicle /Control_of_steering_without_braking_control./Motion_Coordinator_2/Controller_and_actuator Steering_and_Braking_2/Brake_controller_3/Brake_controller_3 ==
  Reference : Inport
  Feedback : Inport  Port=2
  Controller : Subsystem  AncestorBlock=|  DialogController=POWERSYS.PowerSysDialog
      | powerlib_extras/Discrete 
      | Control Blocks/Discrete
      | PI Controller
  Controller1 : Subsystem  AncestorBlock=|  DialogController=POWERSYS.PowerSysDialog
      | powerlib_extras/Discrete 
      | Control Blocks/Discrete
      | PI Controller
  Scope : Scope
  Scope1 : Scope
  Scope2 : Scope  NumInputPorts=2
  Sum1 : Sum  Inputs=-+
  Sum2 : Sum
  Sideslip_Ang : Outport
  Sideslip_Ang1 : Outport  Port=2
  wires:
  Controller/1(Out) -> Scope1/1, Sum2/1, Scope2/1, Sideslip_Ang/1
  Sum1/1 -> Controller/1(Error), Scope/1
  Feedback/1 -> Sum1/1
  Controller1/1(Out) -> Sum2/2
  Reference/1 -> Controller1/1(Error), Sum1/2
  Sum2/1 -> Scope2/2, Sideslip_Ang1/1

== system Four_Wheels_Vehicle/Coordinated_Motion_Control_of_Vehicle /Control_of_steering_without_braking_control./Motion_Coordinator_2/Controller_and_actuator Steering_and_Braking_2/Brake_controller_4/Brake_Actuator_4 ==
  input : Inport
  Actuator : Subsystem
  Cut_off_frequency : Constant  Value=10  SampleTime=-1
  output : Outport
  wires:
  Cut_off_frequency/1 -> Actuator/2(fre)
  Actuator/1(out) -> output/1
  input/1 -> Actuator/1(In1)

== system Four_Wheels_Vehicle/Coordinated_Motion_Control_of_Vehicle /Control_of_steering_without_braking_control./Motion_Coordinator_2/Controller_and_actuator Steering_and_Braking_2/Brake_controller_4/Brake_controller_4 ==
  Reference : Inport
  Feedback : Inport  Port=2
  Controller : Subsystem  AncestorBlock=|  DialogController=POWERSYS.PowerSysDialog
      | powerlib_extras/Discrete 
      | Control Blocks/Discrete
      | PI Controller
  Controller1 : Subsystem  AncestorBlock=|  DialogController=POWERSYS.PowerSysDialog
      | powerlib_extras/Discrete 
      | Control Blocks/Discrete
      | PI Controller
  Scope : Scope
  Scope1 : Scope
  Scope2 : Scope  NumInputPorts=2
  Sum1 : Sum  Inputs=-+
  Sum2 : Sum
  Sideslip_Ang : Outport
  Sideslip_Ang1 : Outport  Port=2
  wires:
  Sum2/1 -> Sideslip_Ang1/1, Scope2/2
  Reference/1 -> Sum1/2, Controller1/1(Error)
  Controller1/1(Out) -> Sum2/2
  Feedback/1 -> Sum1/1
  Sum1/1 -> Scope/1, Controller/1(Error)
  Controller/1(Out) -> Sideslip_Ang/1, Scope2/1, Sum2/1, Scope1/1

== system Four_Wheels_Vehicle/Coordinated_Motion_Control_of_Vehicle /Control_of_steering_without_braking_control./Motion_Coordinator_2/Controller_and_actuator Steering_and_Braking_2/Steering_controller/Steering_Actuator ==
  input : Inport
  Actuator : Subsystem
  Cut_off_frequency : Constant  Value=5  SampleTime=-1
  output : Outport
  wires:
  Cut_off_frequency/1 -> Actuator/2(fre)
  Actuator/1(out) -> output/1
  input/1 -> Actuator/1(In1)

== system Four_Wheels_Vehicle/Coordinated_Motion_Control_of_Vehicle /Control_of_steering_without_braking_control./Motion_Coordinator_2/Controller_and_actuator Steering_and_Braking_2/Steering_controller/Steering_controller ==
  Reference : Inport
  Feedback : Inport  Port=2
  Controller : Subsystem  AncestorBlock=|  DialogController=POWERSYS.PowerSysDialog
      | powerlib_extras/Discrete 
      | Control Blocks/Discrete
      | PI Controller
  Controller1 : Subsystem  AncestorBlock=|  DialogController=POWERSYS.PowerSysDialog
      | powerlib_extras/Discrete 
      | Control Blocks/Discrete
      | PI Controller
  Scope : Scope
  Scope1 : Scope
  Scope2 : Scope  NumInputPorts=2
  Scope3 : Scope  NumInputPorts=2
  Sum1 : Sum  Inputs=-+
  Sum2 : Sum
  Steering_Ang : Outport
  Steering_Ang1 : Outport  Port=2
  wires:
  Feedback/1 -> Sum1/1
  Sum1/1 -> Scope/1, Controller/1(Error)
  Reference/1 -> Scope3/2, Controller1/1(Error), Sum1/2
  Controller/1(Out) -> Sum2/1, Scope2/1, Steering_Ang/1, Scope1/1
  Sum2/1 -> Scope3/1, Scope2/2, Steering_Ang1/1
  Controller1/1(Out) -> Sum2/2

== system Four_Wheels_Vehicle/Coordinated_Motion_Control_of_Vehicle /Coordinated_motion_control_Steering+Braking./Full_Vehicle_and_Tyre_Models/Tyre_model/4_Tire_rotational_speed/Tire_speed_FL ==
  Tb_FL : Inport
  Td_FL : Inport  Port=2
  Fx_FL : Inport  Port=3
  1/Jw : Gain  Gain=1/Jw
  Add22 : Sum  Inputs=-+
  Add23 : Sum  Inputs=+-
  Product27 : Product
  Stop Simulation5 : Stop
  Vx0 : Integrator  InitialCondition=14.3  UpperSaturationLimit=50/3.6  LowerSaturationLimit=eps  ShowSaturationPort=on
  reff : Constant  Value=reff
  Omega_FL : Outport
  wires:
  1/Jw/1 -> Vx0/1
  Tb_FL/1 -> Add22/1
  Td_FL/1 -> Add22/2
  reff/1 -> Product27/2
  Product27/1 -> Add23/2
  Add22/1 -> Add23/1
  Add23/1 -> 1/Jw/1
  Vx0/1 -> Omega_FL/1
  Vx0/2 -> Stop Simulation5/1
  Fx_FL/1 -> Product27/1

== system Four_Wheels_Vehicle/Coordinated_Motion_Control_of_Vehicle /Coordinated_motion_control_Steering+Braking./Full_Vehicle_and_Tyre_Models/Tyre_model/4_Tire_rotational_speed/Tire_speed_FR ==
  Tb_FR : Inport
  Td_FR : Inport  Port=2
  Fx_FR : Inport  Port=3
  1/Jw : Gain  Gain=1/Jw
  Add1 : Sum  Inputs=+-
  Add24 : Sum  Inputs=-+
  Product1 : Product
  Stop Simulation6 : Stop
  Vx1 : Integrator  InitialCondition=14.3  UpperSaturationLimit=50/3.6  LowerSaturationLimit=eps  ShowSaturationPort=on
  reff : Constant  Value=reff
  Omega_FR : Outport
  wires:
  Product1/1 -> Add1/2
  Add1/1 -> 1/Jw/1
  1/Jw/1 -> Vx1/1
  Add24/1 -> Add1/1
  Td_FR/1 -> Add24/2
  Tb_FR/1 -> Add24/1
  reff/1 -> Product1/2
  Fx_FR/1 -> Product1/1
  Vx1/2 -> Stop Simulation6/1
  Vx1/1 -> Omega_FR/1

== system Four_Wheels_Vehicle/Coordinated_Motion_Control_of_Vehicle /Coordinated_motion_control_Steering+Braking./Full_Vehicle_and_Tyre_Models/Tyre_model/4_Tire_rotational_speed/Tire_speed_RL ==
  Tb_RL : Inport
  Td_RL : Inport  Port=2
  Fx_RL : Inport  Port=3
  1/Jw : Gain  Gain=1/Jw
  Add2 : Sum  Inputs=--
  Add22 : Sum  Inputs=-+
  Product2 : Product
  Stop Simulation7 : Stop
  Vx2 : Integrator  InitialCondition=14.3  UpperSaturationLimit=50/3.6  LowerSaturationLimit=eps  ShowSaturationPort=on
  reff : Constant  Value=reff
  Omega_RL : Outport
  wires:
  Fx_RL/1 -> Product2/1
  1/Jw/1 -> Vx2/1
  Vx2/2 -> Stop Simulation7/1
  Vx2/1 -> Omega_RL/1
  reff/1 -> Product2/2
  Product2/1 -> Add2/2
  Add2/1 -> 1/Jw/1
  Add22/1 -> Add2/1
  Tb_RL/1 -> Add22/1
  Td_RL/1 -> Add22/2

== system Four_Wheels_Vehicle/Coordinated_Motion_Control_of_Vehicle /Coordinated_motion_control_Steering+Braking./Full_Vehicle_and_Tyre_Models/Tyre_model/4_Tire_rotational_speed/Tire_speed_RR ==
  Tb_RR : Inport
  Td_RR : Inport  Port=2
  Fx_RR : Inport  Port=3
  1/Jw : Gain  Gain=1/Jw
  Add22 : Sum  Inputs=-+
  Add3 : Sum  Inputs=--
  Product3 : Product
  Stop Simulation8 : Stop
  Vx3 : Integrator  InitialCondition=14.3  UpperSaturationLimit=50/3.6  LowerSaturationLimit=eps  ShowSaturationPort=on
  reff : Constant  Value=reff
  Omega_RR : Outport
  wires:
  Vx3/1 -> Omega_RR/1
  Vx3/2 -> Stop Simulation8/1
  Add3/1 -> 1/Jw/1
  1/Jw/1 -> Vx3/1
  reff/1 -> Product3/2
  Fx_RR/1 -> Product3/1
  Product3/1 -> Add3/2
  Add22/1 -> Add3/1
  Tb_RR/1 -> Add22/1
  Td_RR/1 -> Add22/2

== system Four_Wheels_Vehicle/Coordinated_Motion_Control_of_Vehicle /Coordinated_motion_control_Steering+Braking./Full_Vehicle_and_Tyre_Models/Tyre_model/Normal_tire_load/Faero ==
  note: Air Drag Faero
  Vx : Inport
  AirDragConst1 : Inport  Port=2
  FrontalArea1 : Inport  Port=3
  Airdensity : Inport  Port=4
  windVelocity : Inport  Port=5
  Add : Sum
  Constant : Constant  Value=0.5
  Math Function : Math  Operator=square
  Product : Product  Inputs=5
  Faero : Outport
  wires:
  FrontalArea1/1 -> Product/2
  Constant/1 -> Product/4
  windVelocity/1 -> Add/1
  Add/1 -> Math Function/1
  Math Function/1 -> Product/5
  Product/1 -> Faero/1
  AirDragConst1/1 -> Product/1
  Airdensity/1 -> Product/3
  Vx/1 -> Add/2

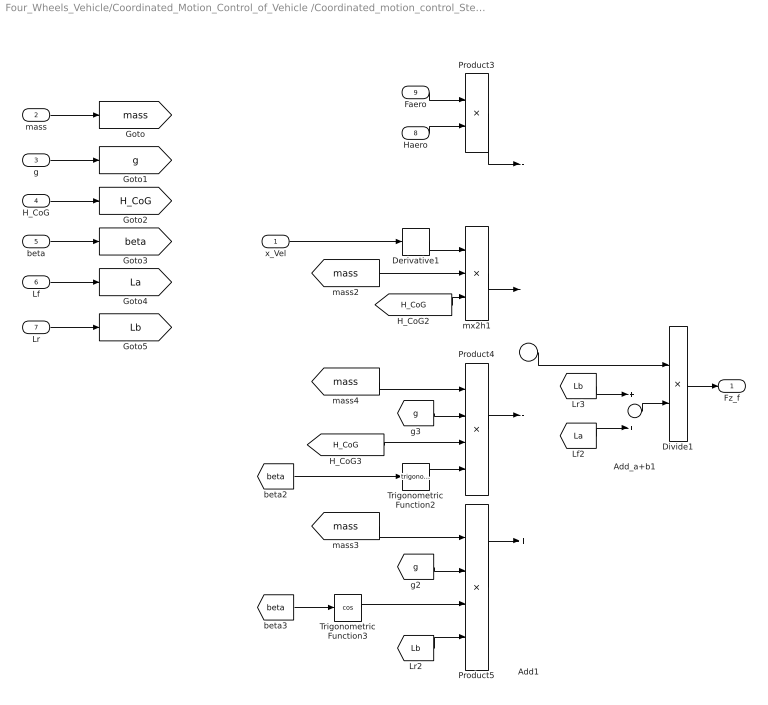
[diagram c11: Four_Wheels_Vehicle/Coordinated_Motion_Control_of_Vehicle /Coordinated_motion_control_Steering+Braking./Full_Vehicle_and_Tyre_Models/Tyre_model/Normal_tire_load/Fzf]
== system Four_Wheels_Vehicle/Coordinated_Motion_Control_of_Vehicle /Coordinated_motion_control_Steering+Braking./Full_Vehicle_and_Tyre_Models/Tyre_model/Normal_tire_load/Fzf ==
  x_Vel : Inport
  mass : Inport  Port=2
  g : Inport  Port=3
  H_CoG : Inport  Port=4
  beta : Inport  Port=5
  Lf : Inport  Port=6
  Lr : Inport  Port=7
  Haero : Inport  Port=8
  Faero : Inport  Port=9
  Add1 : Sum  Inputs=---+
  Add_a+b1 : Sum
  Derivative1 : Derivative
  Divide1 : Product  Inputs=*/
  Product3 : Product
  Product4 : Product  Inputs=4
  Product5 : Product  Inputs=4
  Trigonometric Function2 : Trigonometry
  Trigonometric Function3 : Trigonometry  Operator=cos
  mx2h1 : Product  Inputs=3
  Fz_f : Outport
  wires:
  Derivative1/1 -> mx2h1/1
  [H_CoG] -> mx2h1/3
  [beta] -> Trigonometric Function2/1
  [beta] -> Trigonometric Function3/1
  [H_CoG] -> Product4/3
  Trigonometric Function2/1 -> Product4/4
  [mass] -> Product5/1
  Trigonometric Function3/1 -> Product5/3
  [Lb] -> Product5/4
  [Lb] -> Add_a+b1/1
  [La] -> Add_a+b1/2
  Product3/1 -> Add1/1
  mx2h1/1 -> Add1/2
  Product4/1 -> Add1/3
  Product5/1 -> Add1/4
  Add1/1 -> Divide1/1
  Add_a+b1/1 -> Divide1/2
  Divide1/1 -> Fz_f/1
  x_Vel/1 -> Derivative1/1
  [mass] -> Product4/1
  [g] -> Product4/2
  [mass] -> mx2h1/2
  [g] -> Product5/2
  g/1 -> [g]
  H_CoG/1 -> [H_CoG]
  beta/1 -> [beta]
  Lr/1 -> [Lb]
  Faero/1 -> Product3/1
  Haero/1 -> Product3/2
  mass/1 -> [mass]
  Lf/1 -> [La]

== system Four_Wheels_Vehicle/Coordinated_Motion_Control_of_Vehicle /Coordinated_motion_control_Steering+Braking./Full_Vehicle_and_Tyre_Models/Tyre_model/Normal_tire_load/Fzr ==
  Faero : Inport
  Haero : Inport  Port=2
  xVel : Inport  Port=3
  mass : Inport  Port=4
  g : Inport  Port=5
  HatCG : Inport  Port=6
  beta : Inport  Port=7
  Lf : Inport  Port=8
  Lr : Inport  Port=9
  Add1 : Sum  Inputs=++++
  Add_a+b1 : Sum
  Derivative1 : Derivative
  Divide1 : Product  Inputs=*/
  Product3 : Product
  Product4 : Product  Inputs=4
  Product5 : Product  Inputs=4
  Trigonometric Function2 : Trigonometry
  Trigonometric Function3 : Trigonometry  Operator=cos
  mx2h1 : Product  Inputs=3
  Fzr : Outport
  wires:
  Lr/1 -> [Lb]
  Lf/1 -> [La]
  beta/1 -> [beta]
  HatCG/1 -> [HCG]
  [g] -> Product5/2
  [mass] -> mx2h1/2
  [g] -> Product4/2
  g/1 -> [g]
  [mass] -> Product4/1
  mass/1 -> [mass]
  xVel/1 -> Derivative1/1
  Divide1/1 -> Fzr/1
  Add_a+b1/1 -> Divide1/2
  Add1/1 -> Divide1/1
  Product5/1 -> Add1/4
  Product4/1 -> Add1/3
  mx2h1/1 -> Add1/2
  Product3/1 -> Add1/1
  [La] -> Add_a+b1/2
  [Lb] -> Add_a+b1/1
  [La] -> Product5/4
  Trigonometric Function3/1 -> Product5/3
  [mass] -> Product5/1
  Trigonometric Function2/1 -> Product4/4
  [HCG] -> Product4/3
  [beta] -> Trigonometric Function3/1
  [beta] -> Trigonometric Function2/1
  [HCG] -> mx2h1/3
  Derivative1/1 -> mx2h1/1
  Haero/1 -> Product3/2
  Faero/1 -> Product3/1

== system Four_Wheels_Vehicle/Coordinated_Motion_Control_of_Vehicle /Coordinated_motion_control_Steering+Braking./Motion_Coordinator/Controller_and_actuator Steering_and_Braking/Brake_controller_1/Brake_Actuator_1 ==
  input : Inport
  Actuator : Subsystem
  Cut_off_frequency : Constant  Value=10  SampleTime=-1
  output : Outport
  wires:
  input/1 -> Actuator/1(In1)
  Actuator/1(out) -> output/1
  Cut_off_frequency/1 -> Actuator/2(fre)

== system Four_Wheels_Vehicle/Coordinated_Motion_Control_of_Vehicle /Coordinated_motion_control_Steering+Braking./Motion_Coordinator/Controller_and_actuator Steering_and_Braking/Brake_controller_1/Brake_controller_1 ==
  Reference : Inport
  Feedback : Inport  Port=2
  Controller : Subsystem  AncestorBlock=|  DialogController=POWERSYS.PowerSysDialog
      | powerlib_extras/Discrete 
      | Control Blocks/Discrete
      | PI Controller
  Controller1 : Subsystem  AncestorBlock=|  DialogController=POWERSYS.PowerSysDialog
      | powerlib_extras/Discrete 
      | Control Blocks/Discrete
      | PI Controller
  Scope : Scope
  Scope1 : Scope
  Scope2 : Scope  NumInputPorts=2
  Sum1 : Sum  Inputs=-+
  Sum2 : Sum
  Sideslip_Ang : Outport
  Sideslip_Ang1 : Outport  Port=2
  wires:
  Controller/1(Out) -> Scope1/1, Sum2/1, Scope2/1, Sideslip_Ang/1
  Sum1/1 -> Controller/1(Error), Scope/1
  Feedback/1 -> Sum1/1
  Controller1/1(Out) -> Sum2/2
  Reference/1 -> Controller1/1(Error), Sum1/2
  Sum2/1 -> Scope2/2, Sideslip_Ang1/1

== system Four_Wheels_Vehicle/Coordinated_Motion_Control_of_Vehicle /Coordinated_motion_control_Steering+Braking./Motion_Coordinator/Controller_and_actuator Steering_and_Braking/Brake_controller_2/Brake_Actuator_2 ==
  input : Inport
  Actuator : Subsystem
  Cut_off_frequency : Constant  Value=10  SampleTime=-1
  output : Outport
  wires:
  Cut_off_frequency/1 -> Actuator/2(fre)
  Actuator/1(out) -> output/1
  input/1 -> Actuator/1(In1)
